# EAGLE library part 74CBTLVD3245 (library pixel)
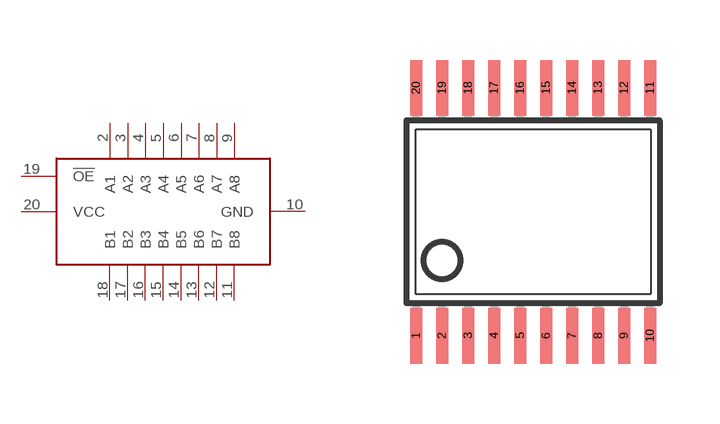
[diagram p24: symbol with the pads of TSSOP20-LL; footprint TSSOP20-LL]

Designator prefix -

## 74CBTLVD3245  [TSSOP20-LL]
2  A1
3  A2
4  A3
5  A4
6  A5
7  A6
8  A7
9  A8
10  GND
11  B8
12  B7
13  B6
14  B5
15  B4
16  B3
17  B2
18  B1
19  !OE
20  VCC

## Footprint TSSOP20-LL (pad centres in mm)
Thin Shrink Small Outline Plastic 20 MAX3223-MAX3243.pdf
smd 0.3 x 1.4: 1 -2.925,-3.1; 2 -2.275,-3.1; 3 -1.625,-3.1; 4 -0.975,-3.1; 5 -0.325,-3.1; 6 0.325,-3.1; 7 0.975,-3.1; 8 1.625,-3.1; 9 2.275,-3.1; 10 2.925,-3.1; 11 2.925,3.1; 12 2.275,3.1; 13 1.625,3.1; 14 0.975,3.1; 15 0.325,3.1; 16 -0.325,3.1; 17 -0.975,3.1; 18 -1.625,3.1; 19 -2.275,3.1; 20 -2.925,3.1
